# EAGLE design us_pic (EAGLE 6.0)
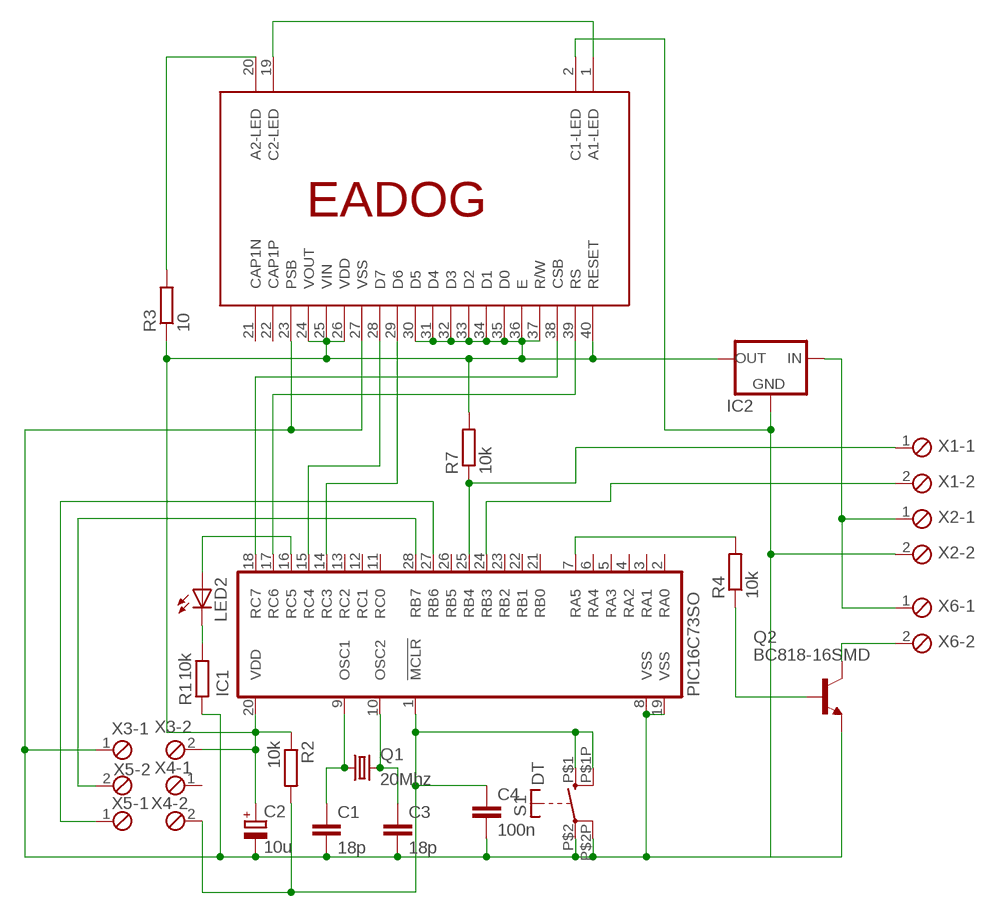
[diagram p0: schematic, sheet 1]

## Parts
C1  18p  C-EUC0805  [C0805]
C2  10u  CPOL-EU153CLV-0605  [153CLV-0605]
C3  18p  C-EUC0805  [C0805]
C4  100n  C-EUC0805  [C0805]
IC1  PIC16C73SO  [SO28W]
IC2  78XXS78XXL_SOT89  [SOT89]
LED2  LEDCHIPLED_1206  [CHIPLED_1206]
Q1  20Mhz  CRYSTALHC49U70  [HC49U70]
Q2  BC818-16SMD  [SOT23-BEC]
R1  10k  R-EU_R1206  [R1206]
R2  10k  R-EU_R1206  [R1206]
R3  10  R-EU_R1206  [R1206]
R4  10k  R-EU_R1206  [R1206]
R7  10k  R-EU_R1206  [R1206]
S1  DT  [DT6]
U$1  EADOG  [EADOG]
X1  MPT2  [2POL254]
X2  MPT2  [2POL254]
X3  MPT2  [2POL254]
X4  MPT2  [2POL254]
X5  MPT2  [2POL254]
X6  MPT2  [2POL254]

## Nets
GND: C1.2 C2.- C3.2 C4.2 IC1.8(VSS) IC1.19(VSS) IC2.2(GND) Q2.E R1.1 S1.P$2(S2) S1.P$2P(S2P) U$1.2(C1-LED) U$1.23(PSB) U$1.27(VSS) X2.2 X3.1
N$1: C1.1 IC1.9(OSC1) Q1.1
N$2: C3.1 IC1.10(OSC2) Q1.2
N$3: LED2.C R1.2
N$4: R3.2 U$1.20(A2-LED)
N$5: IC1.25(RB4) R7.1 X1.1
N$6: C4.1 IC1.1(!MCLR) R2.2 S1.P$1(S1) S1.P$1P(S1P) X4.2
N$7: IC1.28(RB7) X5.2
N$8: IC1.27(RB6) X5.1
N$9: U$1.1(A1-LED) U$1.19(C2-LED)
N$10: Q2.B R4.1
N$11: Q2.C X6.2
N$12: IC1.16(RC5) LED2.A
N$13: IC1.15(RC4) U$1.28(D7)
N$14: IC1.14(RC3) U$1.29(D6)
N$15: IC1.17(RC6) U$1.39(RS)
N$16: IC1.18(RC7) U$1.38(CSB)
N$17: IC1.7(RA5) R4.2
N$18: IC1.24(RB3) X1.2
V+: IC2.3(IN) X2.1 X6.1
VDD: C2.+ IC1.20(VDD) IC2.1(OUT) R2.1 R3.1 R7.2 U$1.24(VOUT) U$1.25(VIN) U$1.26(VDD) U$1.30(D5) U$1.31(D4) U$1.32(D3) U$1.33(D2) U$1.34(D1) U$1.35(D0) U$1.36(E) U$1.37(R/W) U$1.40(RESET) X3.2
Unconnected: IC1.2(RA0) IC1.3(RA1) IC1.4(RA2) IC1.5(RA3) IC1.6(RA4) IC1.11(RC0) IC1.12(RC1) IC1.13(RC2) IC1.21(RB0) IC1.22(RB1) IC1.23(RB2) IC1.26(RB5) U$1.21(CAP1N) U$1.22(CAP1P) X4.1

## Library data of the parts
C1 C3 C4 = resistor:C-EU: CAPACITOR, European symbol
C2 = resistor:CPOL-EU: POLARIZED CAPACITOR, European symbol
IC1 = microchip:PIC16C73: MICROCONTROLLER EPROM/ROM-based; MF: MICROCHIP; MPN: PIC16C73B-20/SO; OC_FARNELL: 9759999; OC_NEWARK: 12C1926
IC2 = Mylib:78XXS: VOLTAGE REGULATOR
LED2 = led:LED: LED
Q1 = crystal:CRYSTAL: CRYSTAL; OC_FARNELL: unknown; OC_NEWARK: unknown
Q2 = Mylib:BC818*: NPN Transistor
R1-R4 R7 = Mylib:R-EU_: RESISTOR, European symbol
S1 = Mylib:DT: ITT SWITCH
U$1 = Mylib:EADOG: LCD Display 2x16
X1-X6 = con-phoenix-254:MPT2: PHOENIX CONNECTOR; OC_FARNELL: unknown; OC_NEWARK: unknown

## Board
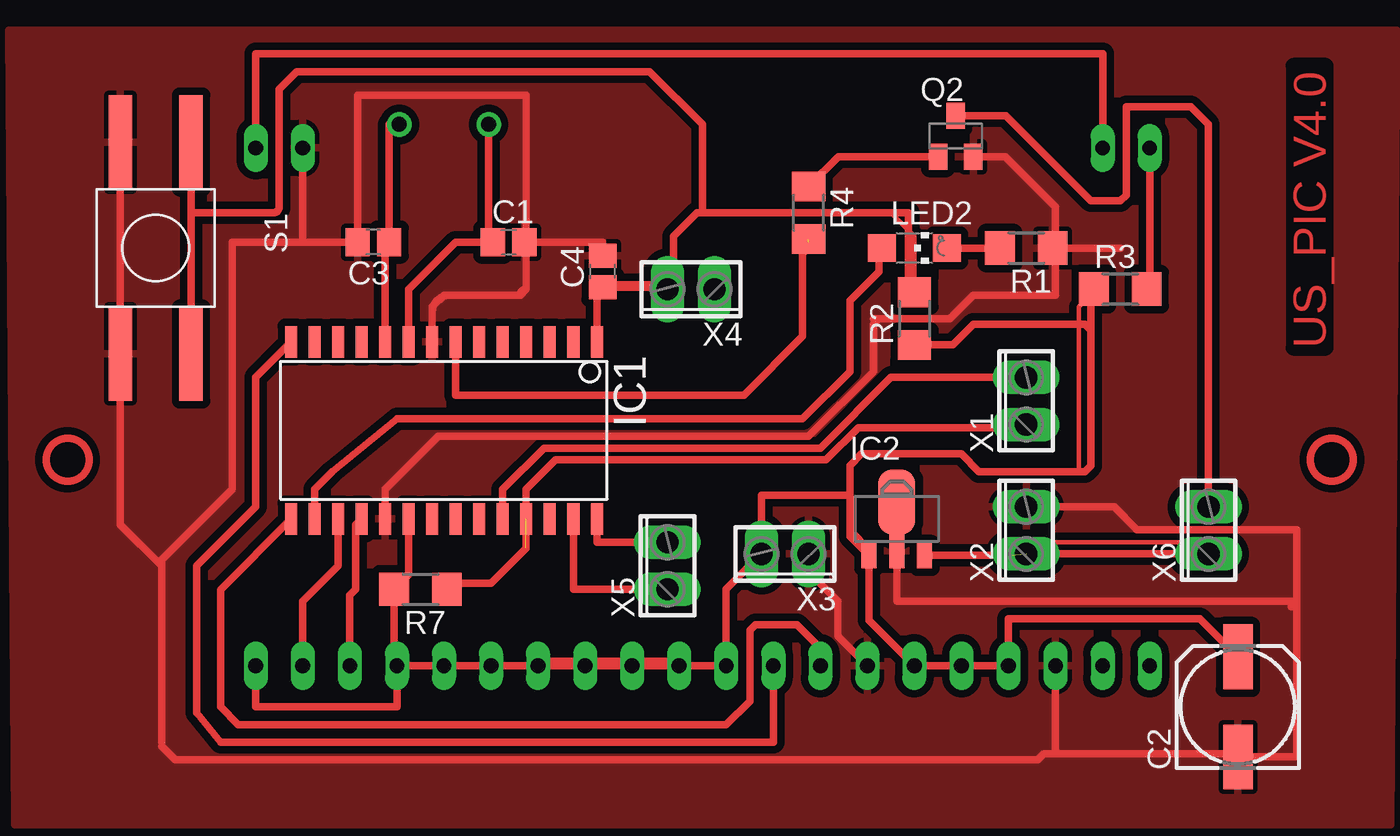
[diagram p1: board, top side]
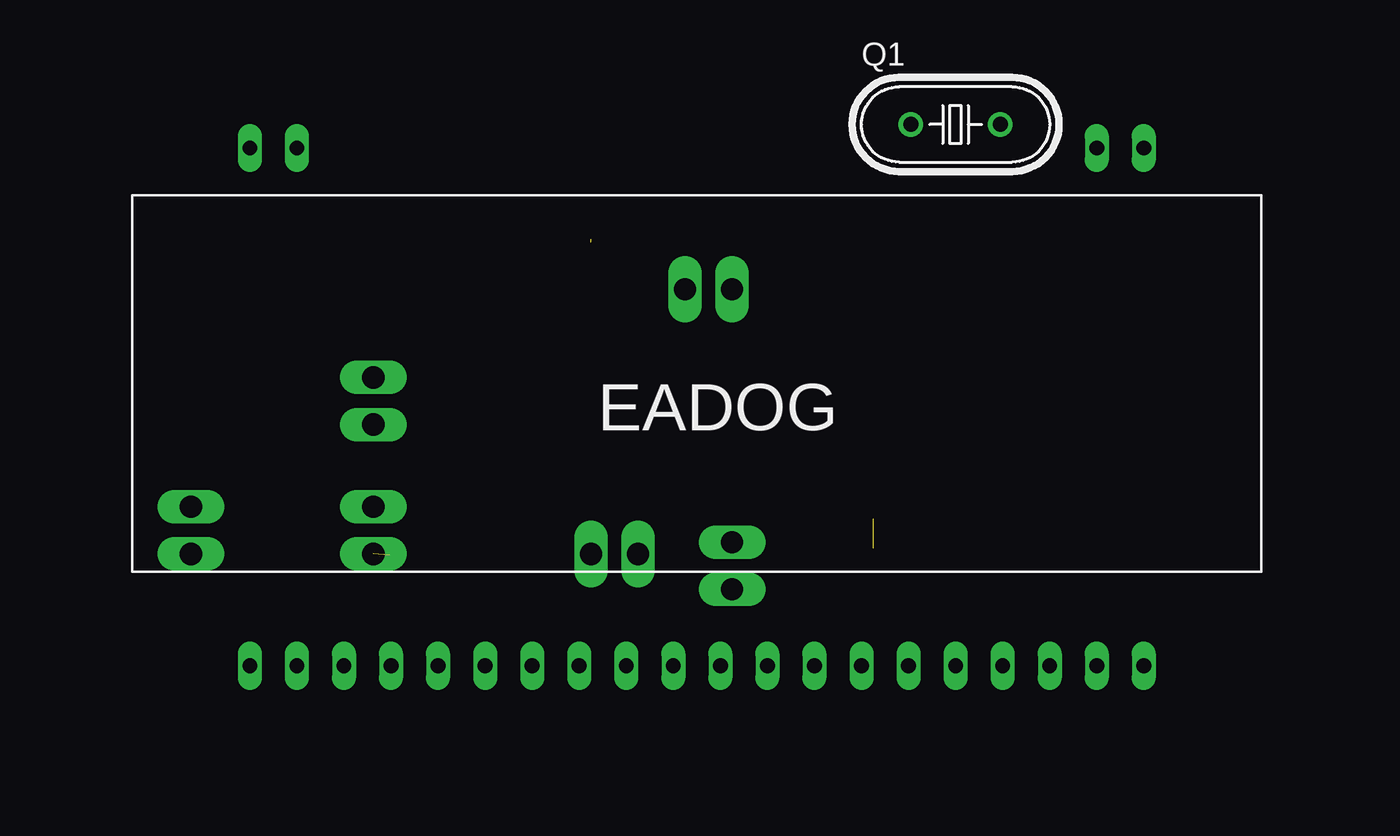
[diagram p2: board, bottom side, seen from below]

No outline drawn. Coordinates in mm, seen from the top.
Copper layers (1*16): Top 0.035mm / dielectric 1.5mm / Bottom 0.035mm
Design rules: minimum track width 10mil, minimum drill 24mil, track to track 8mil, track to pad 8mil, pad to pad 8mil, via to via 8mil, smd to smd 8mil, copper to edge 40mil, drill to drill 8mil, minimum pad ring 10mil, minimum via ring 8mil, stop-mask expansion 4mil, vias tented up to drill 0mil, thermal gap 10mil

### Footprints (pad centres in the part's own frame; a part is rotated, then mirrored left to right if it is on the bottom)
C0805 = smd 1.3 x 1.5: 1 -0.85,0; 2 0.85,0
153CLV-0605 = smd 3.5 x 1.6: + 2.7,0; - -2.7,0
SO28W = smd 0.65 x 1.7: 1 -7.62,-4.78; 2 -6.35,-4.78; 3 -5.08,-4.78; 4 -3.81,-4.78; 5 -2.54,-4.78; 6 -1.27,-4.78; 7 0,-4.78; 8 1.27,-4.78; 9 2.54,-4.78; 10 3.81,-4.78; 11 5.08,-4.78; 12 6.35,-4.78; 13 7.62,-4.78; 14 8.89,-4.78; 15 8.89,4.78; 16 7.62,4.78; 17 6.35,4.78; 18 5.08,4.78; 19 3.81,4.78; 20 2.54,4.78; 21 1.27,4.78; 22 0,4.78; 23 -1.27,4.78; 24 -2.54,4.78; 25 -3.81,4.78; 26 -5.08,4.78; 27 -6.35,4.78; 28 -7.62,4.78
SOT89 = smd 0.8 x 1.4: 1 -1.499,-1.981; 3 1.499,-1.981 | smd 0.8 x 1.9: 2 0,-1.727 | smd 2 x 3.5: 2.1 0,0.889
CHIPLED_1206 = smd 1.5 x 1.5: A 0,-1.75; C 0,1.75
HC49U70 = drill 0.813: 1 -2.413,0; 2 2.413,0
SOT23-BEC = smd 1 x 1.4: B -0.95,-1.1; C 0,1.1; E 0.95,-1.1
R1206 = smd 1.6 x 1.803: 1 -1.422,0; 2 1.422,0
DT6 = smd 5.08 x 1.27: P$1 -6.35,2.54; P$1P 5.08,2.54; P$2 -6.35,-1.27; P$2P 5.08,-1.27
EADOG = drill 0.8 long: 1 -24.13,-10.16; 2 -21.59,-10.16; 19 21.59,-10.16; 20 24.13,-10.16; 21 24.13,17.78; 22 21.59,17.78; 23 19.05,17.78; 24 16.51,17.78; 25 13.97,17.78; 26 11.43,17.78; 27 8.89,17.78; 28 6.35,17.78; 29 3.81,17.78; 30 1.27,17.78; 31 -1.27,17.78; 32 -3.81,17.78; 33 -6.35,17.78; 34 -8.89,17.78; 35 -11.43,17.78; 36 -13.97,17.78; 37 -16.51,17.78; 38 -19.05,17.78; 39 -21.59,17.78; 40 -24.13,17.78
2POL254 = drill 1.2 long: 1 -1.27,0; 2 1.27,0

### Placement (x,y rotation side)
C1  23.81,58.1 0 top
C2  63.18,33.02 90 top
C3  16.51,58.1 180 top
C4  28.89,56.52 90 top
IC1  20.95,47.94 180 top
IC2  44.77,43.18 0 top
LED2  45.72,57.78 270 top
Q1  20.32,64.45 0 bottom
Q2  47.94,63.82 0 top
R1  51.75,57.78 180 top
R2  45.72,53.98 90 top
R3  56.83,55.56 0 top
R4  40.01,59.69 270 top
R7  19.05,39.37 180 top
S1  4.13,57.15 270 top
U$1  34.29,53.02 180 bottom
X1  51.75,49.53 90 top
X2  51.75,42.55 90 top
X3  38.73,41.27 180 top
X4  33.66,55.56 180 top
X5  32.38,40.64 90 top
X6  61.59,42.55 90 top

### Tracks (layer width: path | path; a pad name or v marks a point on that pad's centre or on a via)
GND
  Top 0.406: 19.68,54.29 19.68,54.61 20.32,55.24 20.64,55.24 | 24.77,55.56 24.45,55.24 | 24.77,57.78 24.77,58 C1.2 | 53.34,30.48 63.18,30.48 C2.- 66.36,30.32 66.36,38.42 | C3.2 8.89,58.1 8.89,44.77 5.08,40.96 5.08,40.64 | 19.68,54.29 IC1.8 | 20.64,55.24 arc90 19.68,54.29 | 24.45,55.24 20.64,55.24 | 24.77,55.56 arc90 24.45,55.24 | 24.77,57.78 24.77,55.56 | 25.08,58.1 arc90 24.77,57.78 | 25.08,58.1 24.77,58.1 24.77,66.04 15.66,66.04 C3.2 | 25.08,58.1 28.89,58.1 C4.2 | IC1.19 17.14,44.77 20,47.62 40.01,47.62 43.5,51.12 43.5,53.66 43.81,53.98 | 43.81,53.98 47.62,53.98 48.9,55.24 53.34,55.24 53.34,57.62 R1.1 | 43.81,53.98 43.5,53.98 | X3.1 40.01,40.32 41.59,38.73 41.59,36.83 U$1.27 | 53.34,30.48 U$1.23 | 66.36,38.42 66.36,38.73 | IC2.2 44.77,38.73 66.36,38.73 | 56.83,57.78 R1.1 | 5.08,30.9 5.82,30.16 52.39,30.16 52.7,30.48 53.34,30.48 | U$1.2 12.7,58.1 C3.2 | 51.58,43.81 56.52,43.81 57.74,42.59 66.36,42.59 66.36,38.73 | 66.06,38.42 66.36,38.42 | Q2.E 50.63,62.72 53.34,60.01 53.34,57.95 R1.1 | 5.08,40.64 5.08,31.11 | S1.P$2 2.86,42.86 5.08,40.64
  pour Top (isolate 0.4): -3.17,69.53 -2.86,26.67 71.44,26.67 71.75,69.53
N$1
  Top 0.406: IC1.9 18.41,55.56 20.95,58.1 C1.1 22.73,58.33 Q1.1
N$2
  Top 0.406: IC1.10 17.14,58.1 C3.1 17.36,64.45 Q1.2
N$3
  Top 0.406: LED2.C R1.2
N$4
  Top 0.406: R3.2 58.42,55.73 U$1.20
N$5  (1 unrouted)
  Top 0.406: R7.1 20.79,39.69 22.86,39.69 24.77,41.59 24.77,44.77 26.35,46.35 40.96,46.35 42.7,48.1 51.59,48.1 X1.1
N$6
  Top 0.254: R2.2 45.72,58.42 44.45,59.69 | C4.1 29.21,55.88 31.75,55.88 X4.2
  Top 0.406: 28.57,53.66 IC1.1 28.57,55.66 C4.1 32.6,55.66 32.7,55.56 32.7,58.42 33.97,59.69 34.29,59.69 | 34.29,59.69 44.45,59.69 45.4,59.69 45.4,55.09 | S1.P$1 S1.P$1P | S1.P$1P 6.67,51.75 6.99,51.44 | S1.P$1P 6.67,59.69 11.11,59.69 arc90 11.43,60.01 11.43,66.36 12.38,67.31 31.43,67.31 34.29,64.45 34.29,59.69
N$7
  Top 0.406: IC1.28 28.57,41.91 X5.2
N$8
  Top 0.406: IC1.27 27.3,39.37 X5.1
N$9
  Top 0.406: U$1.19 55.88,68.26 10.16,68.26 U$1.1
N$10
  Top 0.406: R4.1 41.61,62.72 Q2.B
N$11
  Top 0.406: Q2.C 50.65,64.92 55.24,60.33 56.83,60.33 57.15,60.64 57.15,65.41 60.64,65.41 61.59,64.45 X6.2
N$12
  Top 0.406: IC1.16 13.34,44.77 14.29,45.72 17.78,48.58 39.69,48.58 42.23,51.12 42.23,54.93 43.81,56.52 43.81,57.63 LED2.A
N$13
  Top 0.406: IC1.15 8.26,39.35 8.26,33.02 9.21,32.07 35.56,32.07 36.83,33.34 36.83,37.15 37.15,37.47 39.37,37.47 40.64,36.2 U$1.28
N$14
  Top 0.406: IC1.14 10.16,50.82 10.16,43.81 6.99,40.64 6.99,32.7 8.26,31.11 38.1,31.11 U$1.29
N$15
  Top 0.406: U$1.39 12.7,38.73 14.61,40.64 IC1.17
N$16
  Top 0.406: U$1.38 15.24,39.05 15.56,39.37 15.56,42.84 IC1.18
N$17  (1 unrouted)
  Top 0.406: IC1.7 20.95,49.85 36.51,49.85 39.69,53.02 39.69,57.47 40.32,58.1 40.01,58.1
N$18
  Top 0.254: 50.8,50.8 X1.2
  Top 0.406: IC1.24 23.5,44.77 25.72,46.99 40.64,46.99 44.45,50.8 50.8,50.8 51.44,50.8
V+  (1 unrouted)
  Top 0.254: X6.1 60.96,41.91 52.07,41.91 X2.1
  Top 0.406: IC2.3 50.86,41.2 | X2.1 X6.1 61.91,41.27
VDD
  Top 0.254: 54.61,45.72 54.61,54.61 55.88,55.88 R3.1 | 27.94,35.56 25.4,35.56 U$1.34 | 27.94,35.56 30.48,35.56 | 27.94,35.56 U$1.33 | 30.48,35.56 33.02,35.56 U$1.31 | 30.48,35.56 U$1.32
  Top 0.406: U$1.37 18.1,35.56 18.41,35.24 U$1.36 U$1.35 U$1.34 U$1.33 U$1.32 U$1.31 U$1.30 35.56,39.37 X3.2 37.47,44.45 42.23,44.45 | U$1.37 17.63,35.4 R7.2 18.41,40.16 IC1.20 | IC2.1 43.27,37.69 U$1.26 U$1.25 U$1.24 50.8,37.78 61.12,37.78 C2.+ | U$1.40 10.16,33.02 17.78,33.02 U$1.37 | R2.1 47.79,52.55 48.9,53.66 54.93,53.66 55.24,53.34 | 55.24,53.34 55.24,46.04 54.93,45.72 54.61,45.72 49.21,45.72 48.26,46.67 42.86,46.67 42.23,46.04 42.23,44.45 | 42.23,42.55 42.23,44.45 | 42.23,42.55 43.27,41.5 IC2.1 | IC2.1 42.23,42.24 42.23,42.55 | 55.24,55.56 55.24,53.34
(copper drawn outside any net)
  shapes: Top circle x2

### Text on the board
Top: US_PIC V4.0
